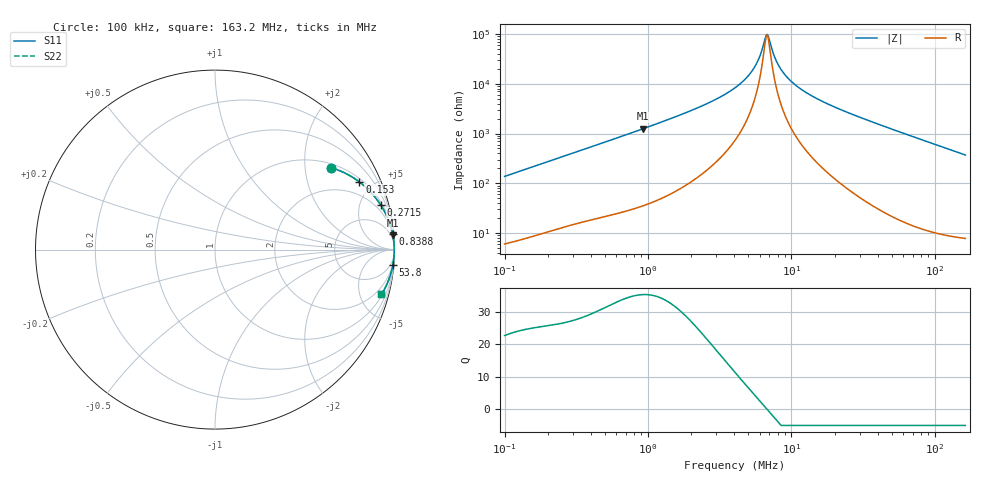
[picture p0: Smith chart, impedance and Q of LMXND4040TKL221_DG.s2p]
! LMXND4040TKL221_DG  S-PARAMETER MODEL  ( General Type )
! Model Generated by TAIYO YUDEN Corporation (http://www.ty-top.com)
! Version 1.0
! TAIYO YUDEN Control No. 191023NI43SB-FBB
! Copyright(c) 2019 TAIYO YUDEN CO.,LTD. All Rights Reserved.
! Product Description (link to TY-COMPAS)
! https://ds.yuden.co.jp/TYCOMPAS/or/detail?pn=LMXND4040TKL221MDG&u=M
! Products Name : Inductors
! Characteristics :
!  Inductance : 220 uH , SRF(min) : 4.0 MHz , DC Resistance(max) : 4.56 Ohm
!  Rated Current : Saturation :275 mA , Temp Rise : 170 mA
!  Case Size : 4.0 x 4.0 / 0.157 x 0.157 [mm/inch] , Thickness : 1.8 / 0.071 [mm/inch]
!  (Conditions: Temperature = 25 degC , DC Bias Current/Voltage = 0A / 0V)
! External Node Assignments :
!  1  o---GGG---o  2
! GND o---------o GND
! Frequency Range : 0.1MHz  -  163.203978MHz  [ 402 STEP ]
# MHz S RI R 50
! Freq[MHz].  S11 Real  S11 Imag  S21 Real  S21 Imag  S12 Real  S12 Imag  S22 Real  S22 Imag
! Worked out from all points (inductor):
!   401 points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, 100 kHz to 163.2 MHz, reference 50 ohm
!   read as one part in series: L = 218 uH near 103.8 kHz
!   highest Q = 35.3 at 920.1 kHz (marker M1), where L = 215 uH
!   self-resonance near 6.656 MHz
!   S11 on the Smith chart (normalised r, x): 100 kHz: 1.12, +2.75; 153 kHz: 1.17, +4.18; 271.5 kHz: 1.27, +7.34; 838.8 kHz: 2, +23; 53.8 MHz: 1, -23; 163.2 MHz: 1.16, -7.40
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0.1  0.6482 0.456  0.3518 -0.456  0.3518 -0.456  0.6482 0.456
0.153014  0.8047 0.3768  0.1953 -0.3768  0.1953 -0.3768  0.8047 0.3768
0.271468  0.923 0.2486  0.077 -0.2486  0.077 -0.2486  0.923 0.2486
0.345249  0.9492 0.2025  0.0508 -0.2025  0.0508 -0.2025  0.9492 0.2025
0.838803  0.9898 0.0874  0.0102 -0.0874  0.0102 -0.0874  0.9898 0.0874
0.920067  0.9913 0.0796  0.00868 -0.0796  0.00868 -0.0796  0.9913 0.0796
1.191969  0.9945 0.061  0.00552 -0.061  0.00552 -0.061  0.9945 0.061
2.5918  0.9982 0.0249  0.00178 -0.0249  0.00178 -0.0249  0.9982 0.0249
4.115259  0.9988 0.0116  0.0012 -0.0116  0.0012 -0.0116  0.9988 0.0116
5.430935  0.9989 0.00493  0.00106 -0.00493  0.00106 -0.00493  0.9989 0.00493
5.957084  0.999 0.00283  0.00104 -0.00283  0.00104 -0.00283  0.999 0.00283
6.534207  0.999 0.000754  0.00102 -0.000754  0.00102 -0.000754  0.999 0.000754
6.780419  0.999 -7.37e-05  0.00102 7.37e-05  0.00102 7.37e-05  0.999 -7.37e-05
7.035908  0.999 -0.000902  0.00102 0.000902  0.00102 0.000902  0.999 -0.000902
7.861604  0.999 -0.0034  0.00103 0.0034  0.00103 0.0034  0.999 -0.0034
8.784198  0.9989 -0.00594  0.00105 0.00594  0.00105 0.00594  0.9989 -0.00594
10.56867  0.9989 -0.0103  0.00113 0.0103  0.00113 0.0103  0.9989 -0.0103
13.94754  0.9987 -0.0177  0.00134 0.0177  0.00134 0.0177  0.9987 -0.0177
22.55928  0.9978 -0.034  0.00224 0.034  0.00224 0.034  0.9978 -0.034
48.15376  0.9925 -0.0776  0.00747 0.0776  0.00747 0.0776  0.9925 -0.0776
53.80481  0.9909 -0.0869  0.00913 0.0869  0.00913 0.0869  0.9909 -0.0869
163.204  0.9274 -0.2492  0.0726 0.2492  0.0726 0.2492  0.9274 -0.2492
